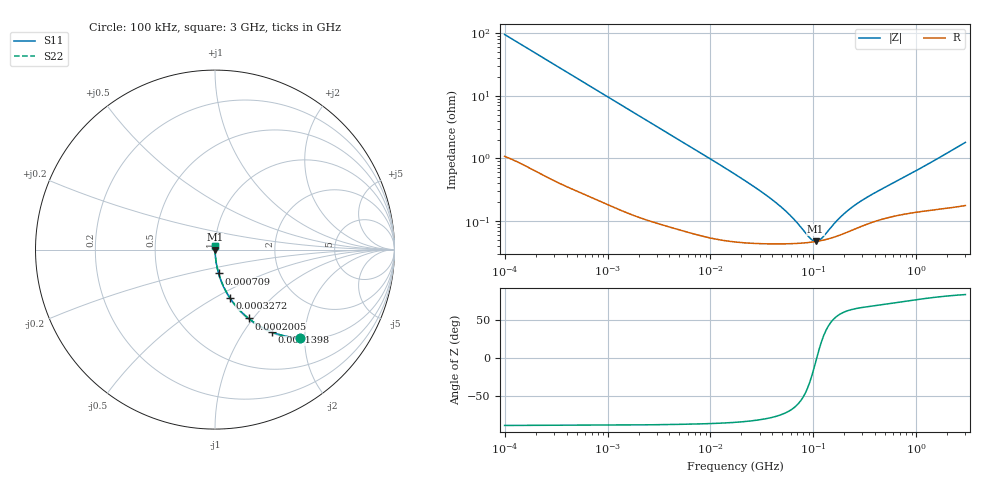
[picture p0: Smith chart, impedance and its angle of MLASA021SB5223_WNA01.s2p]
! MLASA021SB5223_WNA01  S-PARAMETER MODEL  ( Standard Model )
! Model Generated by TAIYO YUDEN Corporation (http://www.ty-top.com)
! Version 1.0
! TAIYO YUDEN Control No. 220901
! Copyright(c) 2022 TAIYO YUDEN CO.,LTD. All Rights Reserved.
! Product Description (link to TY-COMPAS)
! https://ds.yuden.co.jp/TYCOMPAS/or/detail?pn=MLASA021SB5223MWNA01&u=M
! Products Name : Multilayer Ceramic Capacitors
! Characteristics :
!  Capacitance : 0.022 [uF] , Rated Voltage : 4 [V] , TCC : X5R
!  Case Size : 0.25 x 0.125 / 0.0098 x 0.0049 [mm/inch] , Thickness : 0.125 / 0.0049 [mm/inch]
!  (Conditions: Temperature = 25 [degC] , DC Bias Voltage = 0 [V])
! External Node Assignments :
!  1  o---| |---o  2
! GND o---------o GND
! Frequency Range : 100kHz  -  3GHz  [ 401 STEP ]
# MHZ S RI R 50
! Freq[MHz].  S11 Real  S11 Imag  S21 Real  S21 Imag  S12 Real  S12 Imag  S22 Real  S22 Imag
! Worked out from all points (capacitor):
!   401 points, 100 kHz to 3 GHz, reference 50 ohm
!   read as one part in series: C = 16.8 nF near 105.3 kHz
!   lowest |Z| = 47.7 mohm at 105.2 MHz (marker M1)
!   series resonance near 107.7 MHz, so ESL is about 130 pH
!   S11 on the Smith chart (normalised r, x): 100 kHz: 1.02, -1.89; 139.8 kHz: 1.02, -1.36; 200.5 kHz: 1.01, -0.95; 327.2 kHz: 1.01, -0.58; 709 kHz: 1.00, -0.27; 3 GHz: 1.00, +0.04
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0.1  0.4731 -0.4936  0.5269 0.4936  0.5269 0.4936  0.4731 -0.4936
0.1398  0.318 -0.4595  0.682 0.4595  0.682 0.4595  0.318 -0.4595
0.200542  0.1874 -0.3837  0.8126 0.3837  0.8126 0.3837  0.1874 -0.3837
0.327242  0.0819 -0.2672  0.9181 0.2672  0.9181 0.2672  0.0819 -0.2672
0.562235  0.0309 -0.1651  0.9691 0.1651  0.9691 0.1651  0.0309 -0.1651
0.709011  0.0203 -0.1327  0.9797 0.1327  0.9797 0.1327  0.0203 -0.1327
1.385689  0.00631 -0.0694  0.9937 0.0694  0.9937 0.0694  0.00631 -0.0694
3.161081  0.00186 -0.0308  0.9981 0.0308  0.9981 0.0308  0.00186 -0.0308
17.7727  0.000495 -0.00544  0.9995 0.00544  0.9995 0.00544  0.000495 -0.00544
32.15051  0.000446 -0.00282  0.9996 0.00282  0.9996 0.00282  0.000446 -0.00282
48.55934  0.000438 -0.00164  0.9996 0.00164  0.9996 0.00164  0.000438 -0.00164
62.83488  0.000441 -0.00105  0.9996 0.00105  0.9996 0.00105  0.000441 -0.00105
87.84301  0.000457 -0.000379  0.9995 0.000379  0.9995 0.000379  0.000457 -0.000379
97.38194  0.000466 -0.000186  0.9995 0.000186  0.9995 0.000186  0.000466 -0.000186
105.21  0.000474 -4.33e-05  0.9995 4.33e-05  0.9995 4.33e-05  0.000474 -4.33e-05
110.7752  0.000481 5.17e-05  0.9995 -5.17e-05  0.9995 -5.17e-05  0.000481 5.17e-05
119.6798  0.000493 0.000194  0.9995 -0.000194  0.9995 -0.000194  0.000493 0.000194
176.1623  0.000592 0.000918  0.9994 -0.000918  0.9994 -0.000918  0.000592 0.000918
233.9019  0.000714 0.00148  0.9993 -0.00148  0.9993 -0.00148  0.000714 0.00148
326.9943  0.000894 0.0022  0.9991 -0.0022  0.9991 -0.0022  0.000894 0.0022
547.5153  0.00117 0.0036  0.9988 -0.0036  0.9988 -0.0036  0.00117 0.0036
3000  0.0021 0.0179  0.9979 -0.0179  0.9979 -0.0179  0.0021 0.0179
